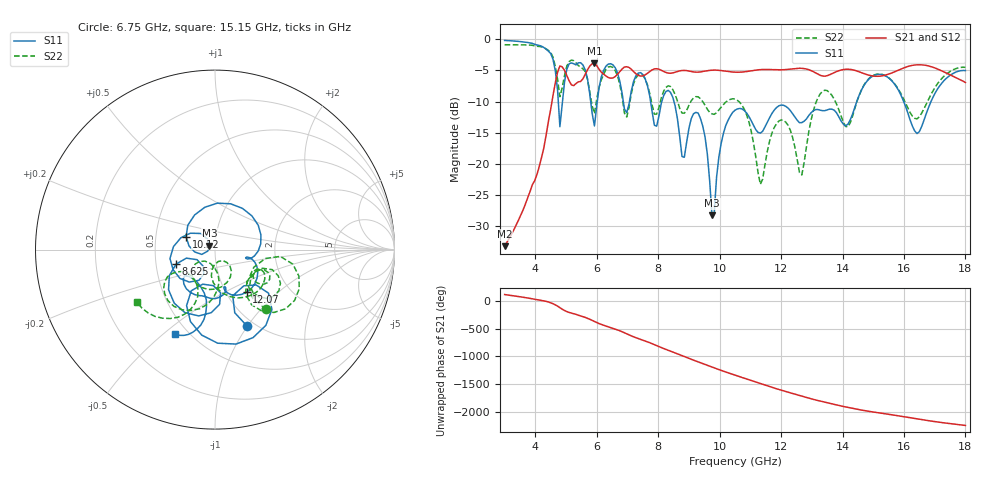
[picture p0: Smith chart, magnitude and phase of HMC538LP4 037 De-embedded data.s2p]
! Chelmsford, MA 01824
! http://www.hittite.com
! Tel: 978-250-3343
! Fax: 978-250-3373
! Device  :  HMC538LP4
! Description:  600 Analog Phase Shifter
! Frequency  :  6.0 GHz - 15.0 GHz
! Package  :  LP4  - 4x4 mm Quad Flatpack No-Lead (QFN) Plastic Package: 24 pin
! Ports  :  2 RF, 1 DC
!  Pin  3  = Rfin  = Port 1
!  Pin  16  = Rfout = Port 2
!  pin  21  = vCTL
! Voltages:  VCTL  = 0 to 5.0 Volts
! Currents :  Vb(V)  Vd(V)  Ib(mA)  Id(mA)
!  0.00  3.70  0.000000	0.473906
! Data:  The device was measured on evaluation board 111296-1.
!  Data was collected using a calibrated network analyzer.
!  The evaluation circuit board was modeled and simulated.This was use
!  to removed the evaluation board circuit from the measured data.
!  The reference plane is the center of the package pin.
! Misc:  Lot #
!Date Measured:  03 - 11 -2009
! Date:  03 - 17 -2009
! Note:
!  Hittite Microwave supplies this data as a sample of measured data at the
!  package pin for this package product.  Your particular data for this product
!  may vary.
!  Data was taken at 25 degrees C.
!  Hittite Microwave reserves the right to change this data at anytime.
# MHz S MA R 50
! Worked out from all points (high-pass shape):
!   201 points, 3 GHz to 18 GHz, reference 50 ohm
!   highest |S21| = -3.87 dB at 5.925 GHz (marker M1); lowest = -33.2 dB at 3 GHz (marker M2)
!   |S21| within 3 dB of the highest: 4.655 GHz to 5.124 GHz (468.6 MHz wide, 9.58 % of centre); 5.391 GHz to 17.98 GHz (12.59 GHz wide, 108 % of centre)
!   lowest |S11| = -28.2 dB at 9.75 GHz (marker M3), VSWR 1.08, Z = 46.9 + j2.14 ohm
!   |S11| at or under -10 dB: 7.752 GHz to 8.118 GHz (365.8 MHz wide, 4.61 % of centre); 8.513 GHz to 14.46 GHz (5.95 GHz wide, 51.8 % of centre); 15.99 GHz to 16.88 GHz (888.3 MHz wide, 5.4 % of centre)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
!   |S22| runs from -23.3 to -0.9 dB; largest |S21 - S12| = 0.0028
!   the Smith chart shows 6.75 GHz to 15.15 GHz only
!   S11 on the Smith chart (normalised r, x): 6.75 GHz: 0.92, -0.99; 8.625 GHz: 0.64, -0.11; 10.12 GHz: 0.72, +0.11; 12.07 GHz: 1.24, -0.65; 15.15 GHz: 0.42, -0.55
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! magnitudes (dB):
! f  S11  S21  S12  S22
! 3 GHz  -0.2  -33.2  -33.2  -0.9
! 4.5 GHz  -2.3  -11.2  -11.2  -2.1
! 4.8 GHz  -14.0  -4.3  -4.3  -9.2
! 5.025 GHz  -4.8  -5.8  -5.9  -4.3
! 5.55 GHz  -4.1  -6.3  -6.4  -4.7
! 5.925 GHz  -13.9  -3.9  -3.9  -11.9
! 6.3 GHz  -4.3  -5.9  -5.9  -4.8
! 6.75 GHz  -6.7  -5.2  -5.2  -7.2
! 8.025 GHz  -12.3  -4.8  -4.8  -10.9
! 8.625 GHz  -12.7  -5.2  -5.2  -9.9
! 9.375 GHz  -12.7  -5.2  -5.2  -9.5
! 9.75 GHz  -28.2  -5.0  -5.0  -12.0
! 10.12 GHz  -15.1  -5.1  -5.1  -10.5
! 10.5 GHz  -11.4  -5.3  -5.3  -9.6
! 11.32 GHz  -15.1  -4.9  -4.9  -23.3
! 12.07 GHz  -10.6  -4.9  -4.9  -13.0
! 12.68 GHz  -13.4  -4.7  -4.7  -21.8
! 13.05 GHz  -11.5  -5.2  -5.2  -11.5
! 15.15 GHz  -5.6  -5.9  -6.0  -5.6
! 15.53 GHz  -6.3  -5.6  -5.6  -6.3
! 16.43 GHz  -15.1  -4.1  -4.1  -12.8
! 18 GHz  -5.0  -6.9  -6.9  -4.5
